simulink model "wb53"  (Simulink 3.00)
settings: Solver=ode113  SolverMode=SingleTasking  StartTime=0.0  StopTime=60  RelTol=1e-3  AbsTol=1e-6

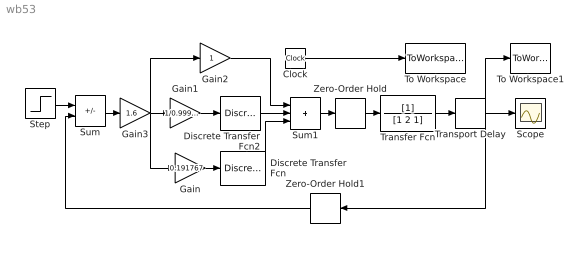
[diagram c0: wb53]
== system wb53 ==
  Clock : Clock
  Discrete Transfer Fcn : DiscreteTransferFcn  Numerator=[1 -1]  Denominator=[1 1]  SampleTime=0.311338
  Discrete Transfer Fcn2 : DiscreteTransferFcn  Numerator=[0.311338 0]  Denominator=[1 -1]  SampleTime=0.311338
  Gain : Gain  Gain=0.191767  SaturateOnIntegerOverflow=on
  Gain1 : Gain  Gain=1/0.9997325  SaturateOnIntegerOverflow=on
  Gain2 : Gain  Gain=1  SaturateOnIntegerOverflow=on
  Gain3 : Gain  Gain=1.6  SaturateOnIntegerOverflow=on
  Scope : Scope
  Step : Step  Time=0  Before=0  After=1  SampleTime=0
  Sum : Sum  Inputs=+-  SaturateOnIntegerOverflow=on
  Sum1 : Sum  Inputs=+++  SaturateOnIntegerOverflow=on
  To Workspace : ToWorkspace  VariableName=t  SampleTime=-1  SaveFormat=Matrix
  To Workspace1 : ToWorkspace  VariableName=y  SampleTime=-1  SaveFormat=Matrix
  Transfer Fcn : TransferFcn  Numerator=[1]  Denominator=[1 2 1]
  Transport Delay : TransportDelay  DelayTime=.5  InitialInput=0  BufferSize=1024
  Zero-Order Hold : ZeroOrderHold  SampleTime=.311338
  Zero-Order Hold1 : ZeroOrderHold  Orientation=left  SampleTime=.311338
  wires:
  Sum1/1 -> Zero-Order Hold/1
  Gain3/1 -> Gain/1, Gain1/1, Gain2/1
  Sum/1 -> Gain3/1
  Zero-Order Hold1/1 -> Sum/2
  Transport Delay/1 -> Zero-Order Hold1/1, To Workspace1/1, Scope/1
  Transfer Fcn/1 -> Transport Delay/1
  Clock/1 -> To Workspace/1
  Step/1 -> Sum/1
  Discrete Transfer Fcn/1 -> Sum1/3
  Gain/1 -> Discrete Transfer Fcn/1
  Gain1/1 -> Discrete Transfer Fcn2/1
  Gain2/1 -> Sum1/1
  Discrete Transfer Fcn2/1 -> Sum1/2
  Zero-Order Hold/1 -> Transfer Fcn/1
